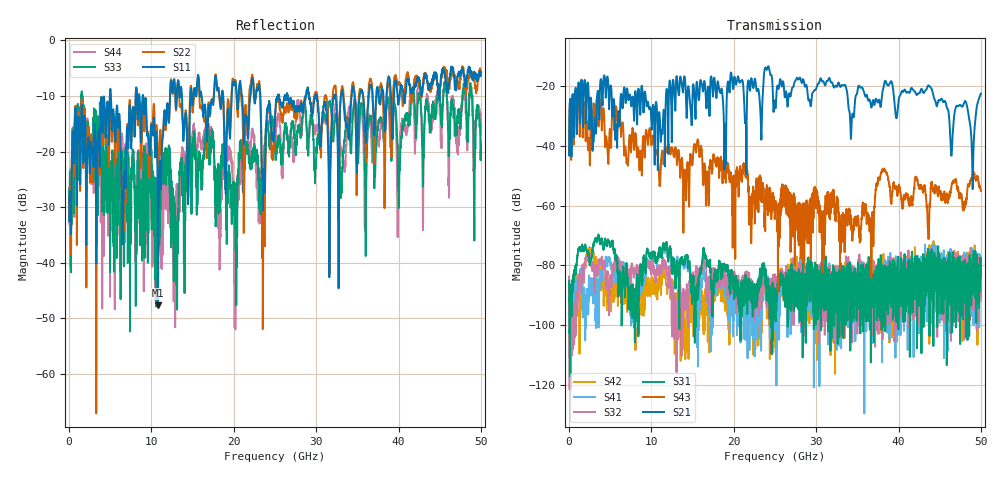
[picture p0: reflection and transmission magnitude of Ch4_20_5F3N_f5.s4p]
!Agilent Technologies,N5247A,US51170199,A.09.90.13
!Agilent N5247A: A.09.90.13
!Date: Monday, December 14, 2015 15:32:17
!Correction: S11(Full 4 Port(1,2,3,4))
!S12(Full 4 Port(1,2,3,4))
!S13(Full 4 Port(1,2,3,4))
!S14(Full 4 Port(1,2,3,4))
!S21(Full 4 Port(1,2,3,4))
!S22(Full 4 Port(1,2,3,4))
!S23(Full 4 Port(1,2,3,4))
!S24(Full 4 Port(1,2,3,4))
!S31(Full 4 Port(1,2,3,4))
!S32(Full 4 Port(1,2,3,4))
!S33(Full 4 Port(1,2,3,4))
!S34(Full 4 Port(1,2,3,4))
!S41(Full 4 Port(1,2,3,4))
!S42(Full 4 Port(1,2,3,4))
!S43(Full 4 Port(1,2,3,4))
!S44(Full 4 Port(1,2,3,4))
!S4P File: Measurements: <S11,S12,S13,S14>,
!<S21,S22,S23,S24>,
!<S31,S32,S33,S34>,
!<S41,S42,S43,S44>:
# Hz S  dB  R 50
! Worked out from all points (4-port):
!   3201 points, 10 MHz to 50 GHz, reference 50 ohm
!   strongest paths, dB at 10 MHz, 12.51 GHz, 25 GHz, 37.5 GHz, 50 GHz:
!     S21: -43.3, -27.9, -26.1, -25.6, -22.6
!     S43: -43.1, -40.7, -59.9, -52.2, -55.1
!     S31: -85.1, -82.1, -90.7, -81.9, -80.6
!     S32: -83.7, -91.8, -86.2, -102.8, -78.5
!     S41: -84.9, -78.0, -87.7, -83.8, -82.9
!     S42: -89.0, -87.9, -97.0, -86.3, -91.8
!   lowest |S11| = -47.7 dB at 10.8 GHz (marker M1), VSWR 1.01, Z = 50 + j0.41 ohm
!   |S11| at or under -10 dB: start of sweep to 4.951 GHz; 5.089 GHz to 8.083 GHz (2.995 GHz wide, 45.5 % of centre); 8.995 GHz to 12.26 GHz (3.264 GHz wide, 30.7 % of centre)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
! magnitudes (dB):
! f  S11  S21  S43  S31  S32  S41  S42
! 10 MHz  -32.6  -43.3  -43.1  -85.1  -83.7  -84.9  -89.0
! 4.087 GHz  -16.3  -24.2  -28.7  -72.9  -80.0  -80.3  -81.6
! 10.8 GHz  -47.7  -40.9  -44.7  -76.2  -81.9  -76.8  -86.4
! 12.59 GHz  -9.3  -18.9  -41.4  -80.1  -95.2  -77.2  -85.4
! 24.04 GHz  -12.4  -14.6  -57.9  -86.4  -86.9  -86.9  -89.7
! 48.98 GHz  -7.1  -52.7  -49.5  -82.1  -77.2  -90.6  -78.5
! 50 GHz  -5.7  -22.6  -55.1  -80.6  -78.5  -82.9  -91.8
